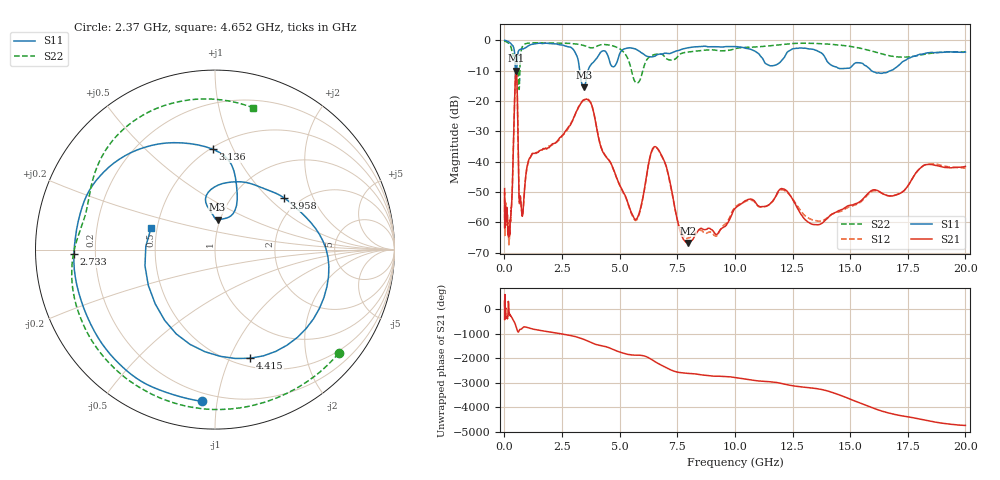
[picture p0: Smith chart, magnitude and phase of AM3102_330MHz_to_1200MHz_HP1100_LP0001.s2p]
! Date/Time: Tue, Sep 11, 2018 5:20 PM
! Network Analyzer: Agilent Technologies E8362B Rev: A.07.50.63
! Sweep from 0.010 to 20.000 GHz, 1601 Points, Sweep Type: LOG
! Power Supply: 4.949 V, 0.001 A
# Hz S DB R 50
!freq MagS11 AngS11 MagS21 AngS21 MagS12 AngS12 MagS22 AngS22
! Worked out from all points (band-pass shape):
!   1601 points, 10 MHz to 20 GHz, reference 50 ohm
!   highest |S21| = -10.07 dB at 508.4 MHz (marker M1); lowest = -66.8 dB at 7.958 GHz (marker M2)
!   |S21| within 3 dB of the highest: 473.1 MHz to 543.1 MHz (69.98 MHz wide, 13.8 % of centre)
!   lowest |S11| = -15.6 dB at 3.449 GHz (marker M3), VSWR 1.40, Z = 48.6 + j16.6 ohm
!   |S11| at or under -10 dB: 472.1 MHz to 532.2 MHz (60.09 MHz wide, 12 % of centre); 3.268 GHz to 3.628 GHz (360 MHz wide, 10.4 % of centre); 15.92 GHz to 16.77 GHz (850.2 MHz wide, 5.2 % of centre)
!   |S22| runs from -16.2 to -0.2 dB; largest |S21 - S12| = 0.0051
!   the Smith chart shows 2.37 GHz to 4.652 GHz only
!   S11 on the Smith chart (normalised r, x): 2.37 GHz: 0.15, -0.91; 2.733 GHz: 0.12, -0.01; 3.136 GHz: 0.51, +0.84; 3.958 GHz: 1.66, +1.25; 4.415 GHz: 0.59, -1.19; 4.652 GHz: 0.46, +0.13
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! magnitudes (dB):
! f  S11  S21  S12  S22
! 10 MHz  -0.1  -48.9  -62.1  -0.2
! 35.55 MHz  -0.1  -57.7  -59.7  -0.3
! 126.4 MHz  -0.3  -58.6  -59.1  -0.7
! 192.9 MHz  -0.5  -63.9  -66.7  -1.0
! 290.2 MHz  -1.2  -56.2  -56.9  -2.3
! 447.2 MHz  -4.5  -18.8  -18.8  -4.3
! 508.4 MHz  -13.0  -10.1  -10.1  -9.2
! 556.4 MHz  -7.2  -16.5  -16.6  -11.3
! 641.7 MHz  -3.2  -52.6  -53.0  -16.1
! 768.6 MHz  -2.8  -57.9  -57.6  -2.3
! 1.59 GHz  -1.0  -36.2  -36.2  -0.8
! 2.37 GHz  -1.4  -32.4  -32.8  -0.9
! 2.733 GHz  -2.1  -29.1  -29.5  -1.0
! 3.136 GHz  -5.0  -23.4  -23.4  -1.2
! 3.449 GHz  -15.6  -19.7  -19.7  -1.7
! 3.958 GHz  -6.4  -27.1  -27.0  -2.1
! 4.415 GHz  -3.9  -38.5  -38.4  -1.4
! 4.652 GHz  -8.5  -41.1  -41.1  -1.7
! 5.652 GHz  -2.8  -58.9  -59.2  -13.5
! 6.612 GHz  -4.8  -35.4  -35.5  -4.6
! 7.958 GHz  -2.5  -66.8  -65.3  -3.9
! 20 GHz  -3.9  -41.6  -42.1  -3.8
